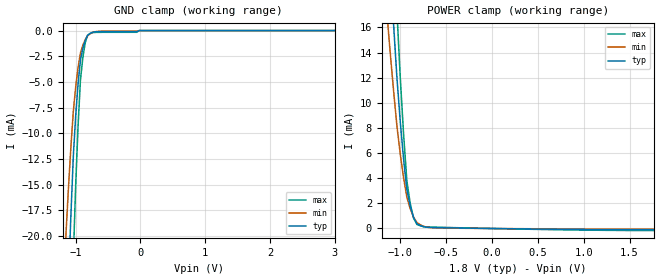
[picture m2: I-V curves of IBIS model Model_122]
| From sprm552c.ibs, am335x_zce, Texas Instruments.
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| Model based on original model for IQ18HYENPB_SSBHH
|   Sub model ENPB_SSBHH_PU_ON_1P8
[model]   Model_122
|[Description]  [1.8V-INPUT-PU-X]
|   Weak internal pull-up, ,
|[Input Load]   PU
|[Output Drive]
|Voltage   1.8V
|Mode   INPUT
Model_type   Input
Polarity   Non-Inverting
Vinl =  0.63
Vinh =  1.17
C_comp   0.9817759p   0.8451655p   1.124986p
[Model Spec]
Vinl   0.63   0.567   0.6615
Vinh   1.17   1.053   1.2285
[Temperature Range]   25   125   -40
[Voltage Range]   1.8   1.62   1.89
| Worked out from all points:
|   GND clamp passes 1 mA (typ) near -0.86 V on its own axis
|   POWER clamp passes 1 mA (typ) near -0.86 V on its own axis
[POWER_clamp]
-1.8V     125.4mA    90.81mA    173.8mA
-1.145V   25.47mA    17.23mA    36.77mA
-1.109V   20.78mA    14.02mA    30.06mA
-1.073V   16.32mA    11.02mA    23.62mA
-1.036V   12.09mA    8.214mA    17.42mA
-1V       8.569mA    5.965mA    12.12mA
-963.6mV  5.566mA    4.055mA    7.578mA
-927.3mV  3.084mA    2.484mA    3.798mA
-854.5mV  878.5uA    907.7uA    836.5uA
-818.2mV  387.5uA    476.2uA    326.5uA
-600mV    68.13uA    44.01uA    102.1uA
1.764V    -96.73uA   -46.42uA   -163.5uA
[GND_clamp]
-1.8V     -191.2mA   -126.8mA   -307.3mA
-1.145V   -30.73mA   -19.2mA    -53.52mA
-1.109V   -23.89mA   -14.96mA   -41.99mA
-1.073V   -17.69mA   -11.16mA   -31.46mA
-1.036V   -12.15mA   -7.794mA   -21.93mA
-1V       -8.265mA   -5.454mA   -14.97mA
-963.6mV  -5.174mA   -3.584mA   -9.276mA
-927.3mV  -2.872mA   -2.184mA   -4.839mA
-890.9mV  -1.761mA   -1.446mA   -2.681mA
-854.5mV  -964.5uA   -891.8uA   -1.219mA
-781.8mV  -295.7uA   -335.4uA   -294.6uA
3.6V      0A         0A         0A
